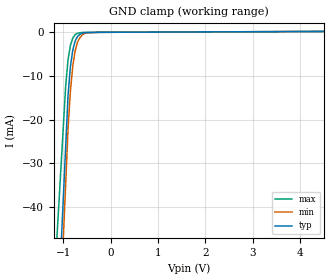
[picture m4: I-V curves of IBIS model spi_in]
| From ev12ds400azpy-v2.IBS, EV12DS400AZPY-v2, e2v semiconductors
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[Model] spi_in
Model_type Input
Vinl = 800.000mV
Vinh = 1.60000V
C_comp 487.000fF 449.000fF 525.000fF
| variable typ   min   max
[Voltage Range] 3.30000V 3.15000V 3.45000V
[POWER Clamp Reference] 3.30000V 3.15000V 3.45000V
[GND Clamp Reference] 0.00000V 0.00000V 0.00000V
[Temperature Range]   25   110   -40
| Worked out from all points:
|   GND clamp passes 1 mA (typ) near -0.70 V on its own axis
[GND Clamp]
-3.3V     -578.3mA   -624.1mA   -452.8mA
-950mV    -26.27mA   -34.77mA   -12.35mA
-900mV    -14.52mA   -22.23mA   -6.361mA
-850mV    -7.891mA   -13.53mA   -3.073mA
-800mV    -4.133mA   -7.776mA   -1.399mA
-750mV    -2.076mA   -4.292mA   -601.8uA
-700mV    -1.017mA   -2.324mA   -267.2uA
-650mV    -526.4uA   -1.303mA   -182.2uA
-600mV    -262.2uA   -674.6uA   -97.27uA
-550mV    -145.9uA   -352.6uA   -92.78uA
-250mV    -67.63uA   -68.83uA   -68.28uA
6.6V      218.2uA    220.2uA    211.9uA
[POWER Clamp]
-3.3V     0A         0A         0A
6.6V      0A         0A         0A
